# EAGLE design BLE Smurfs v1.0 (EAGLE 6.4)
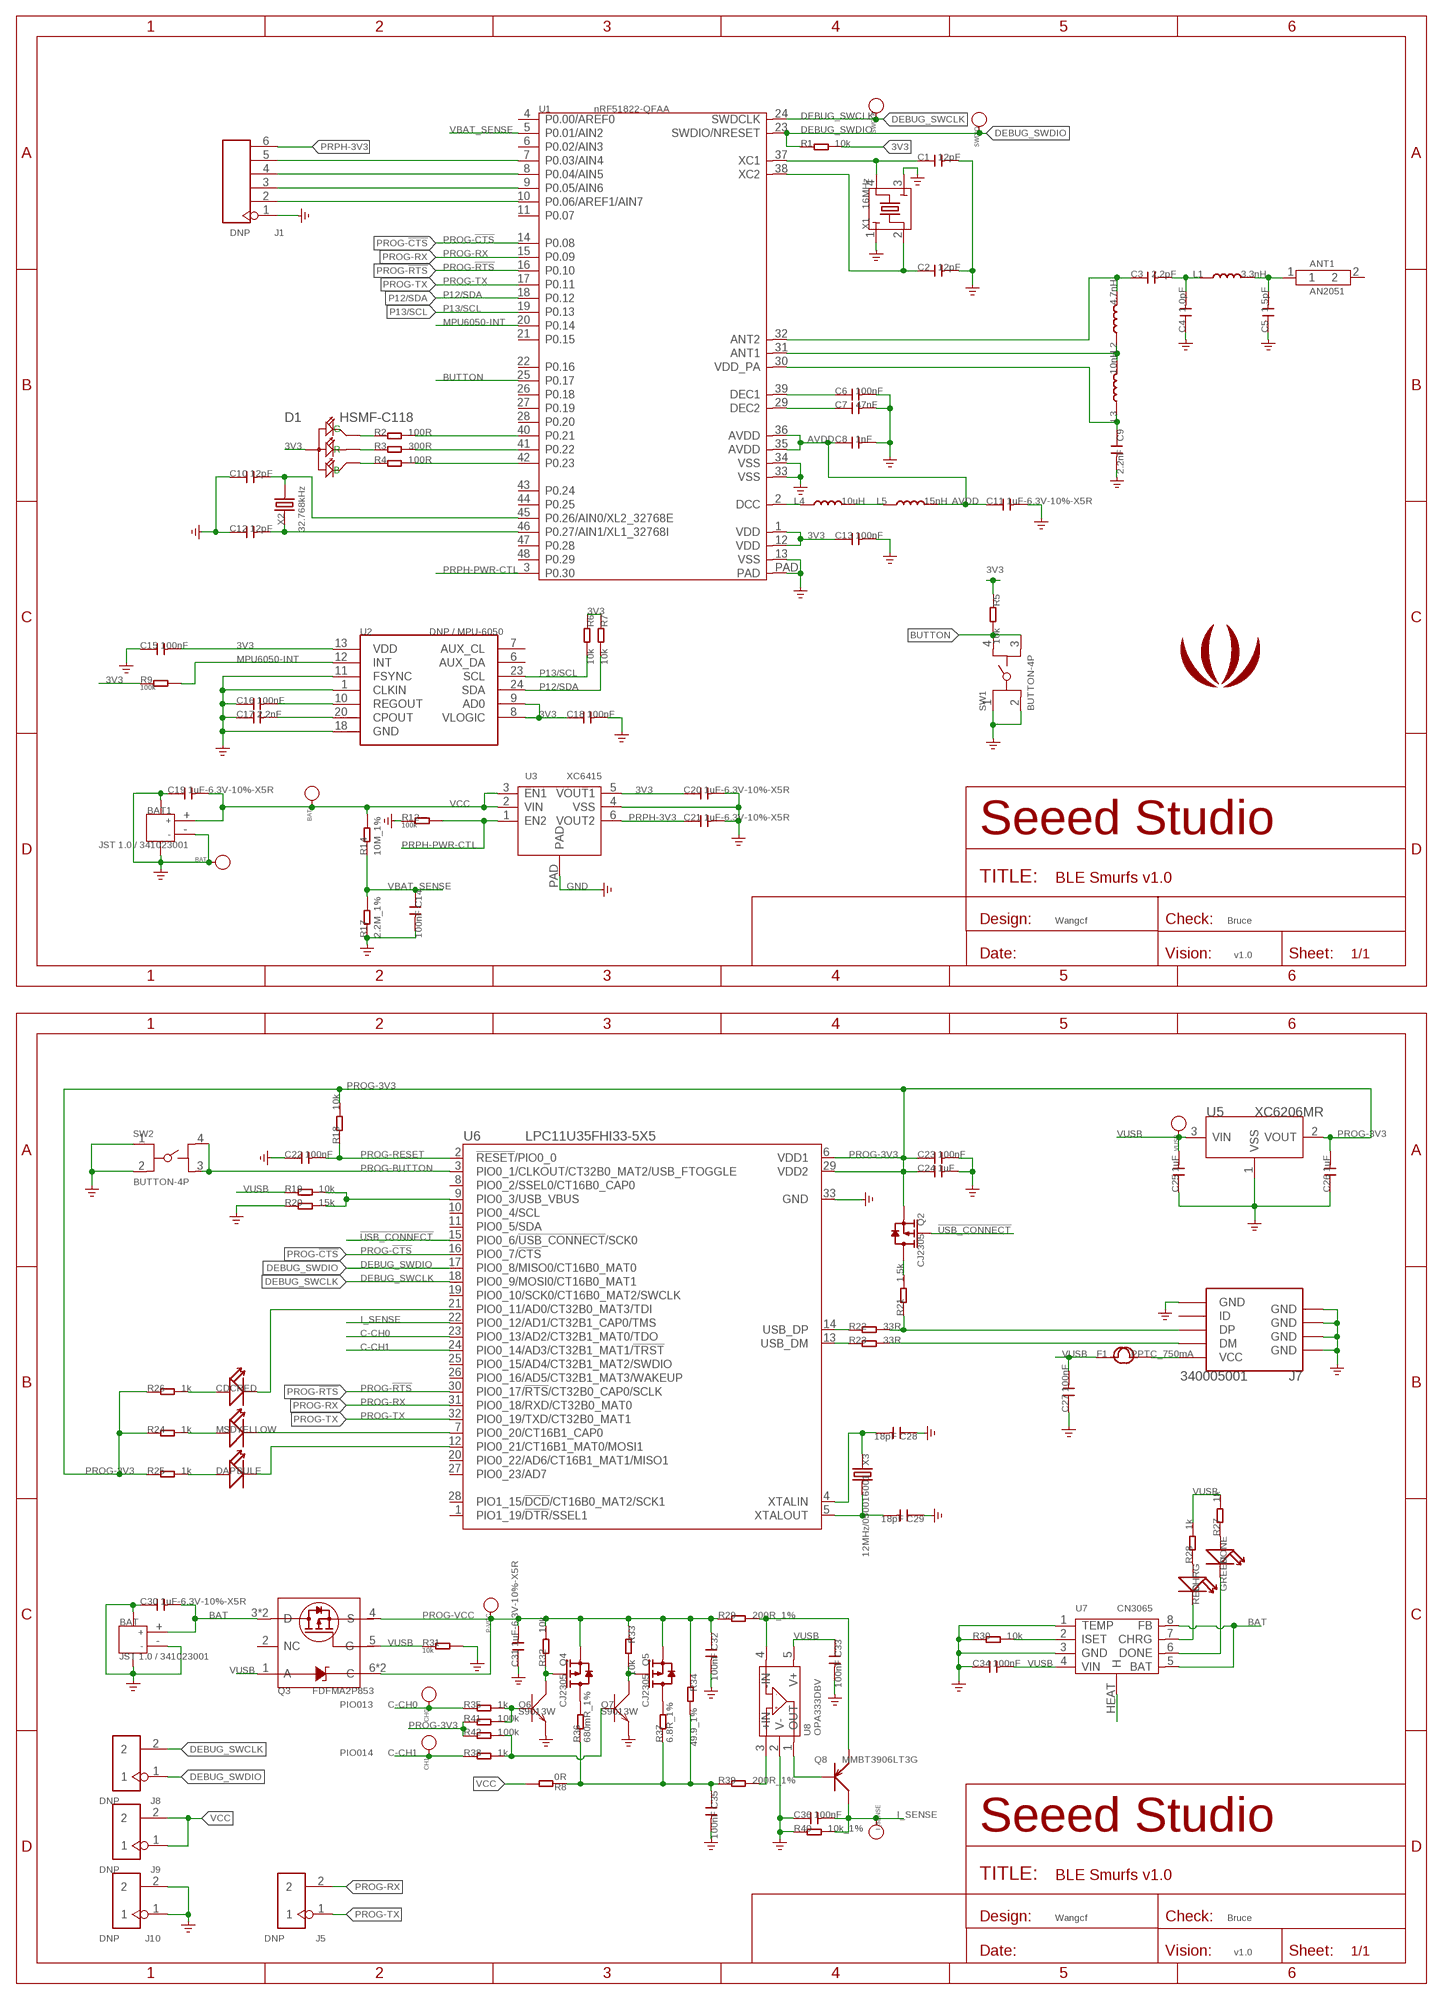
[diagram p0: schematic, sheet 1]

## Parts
ANT1  AN2051  ANTENNA-2.4GHZ-0.5DBI'AN2051'  [2P-SMD-L5.05*W.02*H1.07MM]
BAT  JST 1.0 / 341023001  JACK-JST-2P-SMD-PW'1.0'  [JST-SMD-2P-1.0-90D]
BAT1  JST 1.0 / 341023001  JACK-JST-2P-SMD-PW'1.0'  [JST-SMD-2P-1.0-90D]
BAT+  BAT+  PAD-TEST-POINT'4080'  [PAD_4080]
BAT-  BAT-  PAD-TEST-POINT'4080'  [PAD_4080]
C1  12pF  C-0402  [C0402]
C2  12pF  C-0402  [C0402]
C3  2.2pF  C-0402  [C0402]
C4  1.0pF  C-0402  [C0402]
C5  1.5pF  C-0402  [C0402]
C6  100nF  C-0402  [C0402]
C7  47nF  C-0402  [C0402]
C8  1nF  C-0402  [C0402]
C9  2.2nF  C-0402  [C0402]
C10  12pF  C-0402  [C0402]
C11  1uF-6.3V-10%-X5R  C-0402  [C0402]
C12  12pF  C-0402  [C0402]
C13  100nF  C-0402  [C0402]
C14  100nF  C-0402  [C0402]
C15  100nF  C-0402  [C0402]
C16  100nF  C-0402  [C0402]
C17  2.2nF  C-0402  [C0402]
C18  100nF  C-0402  [C0402]
C19  1uF-6.3V-10%-X5R  C-0402  [C0402]
C20  1uF-6.3V-10%-X5R  C-0402  [C0402]
C21  1uF-6.3V-10%-X5R  C-0402  [C0402]
C22  100nF  C-0402  [C0402]
C23  100nF  C-0402  [C0402]
C24  1uF  C-0402  [C0402]
C25  1uF  C-0402  [C0402]
C26  1uF  C-0402  [C0402]
C27  100nF  C-0402  [C0402]
C28  18pF  C-0402  [C0402]
C29  18pF  C-0402  [C0402]
C30  1uF-6.3V-10%-X5R  C-0402  [C0402]
C31  1uF-6.3V-10%-X5R  C-0402  [C0402]
C32  100nF  C-0402  [C0402]
C33  100nF  C-0402  [C0402]
C34  100nF  C-0402  [C0402]
C35  100nF  C-0402  [C0402]
C36  100nF  C-0402  [C0402]
CDC  RED  LED'0603'  [LED-0603]
CH0  CH0  PAD-TEST-POINT'4545'  [TP_4545]
CH1  CH1  PAD-TEST-POINT'4545'  [TP_4545]
CHRG  RED  LED'0603'  [LED-0603]
D1  HSMF-C118  LED-ARGB-4P-1210  [LED-4P-1210-3.0X2.54]
DAP  BULE  LED'0603'  [LED-0603]
DONE  GREEN  LED'0603'  [LED-0603]
F1  PPTC_750mA  FUSE'1206'  [F1206]
I_SENSE  I_SENSE  PAD-TEST-POINT'4545'  [TP_4545]
J1  DNP  HEADER-6P-60/35MIL  [6P-2.54-60/35MIL]
J5  DNP  HEADER-2P-65/35MIL  [2P-2.54-65/35MIL]
J7  340005001  USB-MINIUSB-5P-MICRO  [MICRO-USB]
J8  DNP  HEADER-2P-65/35MIL  [2P-2.54-65/35MIL]
J9  DNP  HEADER-2P-65/35MIL  [2P-2.54-65/35MIL]
J10  DNP  HEADER-2P-65/35MIL  [2P-2.54-65/35MIL]
L1  3.3nH  L'0402'  [L0402]
L2  4.7nH  L'0402'  [L0402]
L3  10nH  L'0402'  [L0402]
L4  10uH  L'0603'  [L0603]
L5  15nH  L'0402'  [L0402]
MSD  YELLOW  LED'0603'  [LED-0603]
P-VCC  P_VCC  PAD-TEST-POINT'4545'  [TP_4545]
Q2  CJ2305  MOSFET-P'SI2323CDS/SI2305DS<BR>'  [SOT23]
Q3  FDFMA2P853  [6P-SMD-W/-HEAT]
Q4  CJ2305  MOSFET-P'SI2323CDS/SI2305DS<BR>'  [SOT23]
Q5  CJ2305  MOSFET-P'SI2323CDS/SI2305DS<BR>'  [SOT23]
Q6  S9013W  TRANSISTOR-NPN-SOT323  [SOT323]
Q7  S9013W  TRANSISTOR-NPN-SOT323  [SOT323]
Q8  MMBT3906LT3G  TRANSISTOR-PNP-SOT23  [SOT23]
R1  10k  R-0402  [R0402]
R2  100R  R-0402  [R0402]
R3  300R  R-0402  [R0402]
R4  100R  R-0402  [R0402]
R5  10k  R-0402  [R0402]
R6  10k  R-0402  [R0402]
R7  10k  R-0402  [R0402]
R8  0R  R-0603  [R0603]
R9  100k  R-0402  [R0402]
R12  100k  R-0402  [R0402]
R14  10M_1%  R-0402  [R0402]
R17  2.2M_1%  R-0402  [R0402]
R18  10k  R-0402  [R0402]
R19  10k  R-0402  [R0402]
R20  15k  R-0402  [R0402]
R21  1.5k  R-0402  [R0402]
R22  33R  R-0402  [R0402]
R23  33R  R-0402  [R0402]
R24  1k  R-0402  [R0402]
R25  1k  R-0402  [R0402]
R26  1k  R-0402  [R0402]
R27  1k  R-0402  [R0402]
R28  1k  R-0402  [R0402]
R29  200R_1%  R-0402  [R0402]
R30  10k  R-0402  [R0402]
R31  10k  R-0402  [R0402]
R32  10k  R-0402  [R0402]
R33  10k  R-0402  [R0402]
R34  49.9_1%  R-0603  [R0603]
R35  1k  R-0402  [R0402]
R36  680mR_1%  R-0603  [R0603]
R37  6.8R_1%  R-0603  [R0603]
R38  1k  R-0402  [R0402]
R39  200R_1%  R-0402  [R0402]
R40  10k_1%  R-0402  [R0402]
R41  100k  R-0402  [R0402]
R42  100k  R-0402  [R0402]
SW1  BUTTON-4P  [4P-SMD-L4.45*W3.22*H2.5MM]
SW2  BUTTON-4P  [4P-SMD-L4.45*W3.22*H2.5MM]
SWCLK  SWDCLK  PAD-TEST-POINT'4080'  [PAD_4080]
SWDIO  SWDIO  PAD-TEST-POINT'4080'  [PAD_4080]
U1  nRF51822-QFAA  NRF51822  [QFN48-6X6MM]
U2  DNP / MPU-6050  MPU-6050‘’  [QFN24]
U3  XC6415  [USP-6C]
U5  XC6206MR  [SOT23]
U6  LPC11U35FHI33-5X5  [HVQFN33]
U7  CN3065  PMIC-CN3065-DFN8  [DFN-8]
U8  OPA333DBV  [SOT23-5]
U$59  LOGO-SEEEDSTUDIO-SMALL-SILK  [SMALL_SEEED_LOGO]
VUSB  VUSB  PAD-TEST-POINT'4545'  [TP_4545]
X1  16MHz  CRYSTAL'-2520'  [2520]
X2  32.768kHz  CRYSTAL-3215  [2P-SMD-3.2X1.5]
X3  12MHz/050016001  CRYSTAL'5032'  [2P-SMD-5X3.2]

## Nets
3V3: C13.1 C15.2 C18.1 C20.1 D1.1(+) R1.2 R5.1 R6.1 R7.1 R9.1 U1.1(VDD) U1.12(VDD) U2.8(VLOGIC) U2.9(AD0) U2.13(VDD) U3.5(VOUT1)
!USB_CONNECT: Q2.1(G) U6.15(PIO0_6/!USB_CONNECT!/SCK0)
AVDD: C8.1 C11.1 L5.2 U1.35(AVDD) U1.36(AVDD)
BAT: BAT.+ C30.2 Q3.3(D) Q3.P2(D) U7.5(BAT) U7.8(FB)
BUTTON: R5.2 SW1.3 SW1.4 U1.25(P0.17)
C-CH0: CH0.T R35.1 U6.23(PIO0_13/AD2/CT32B1_MAT0/TDO)
C-CH1: CH1.T R38.1 U6.24(PIO0_14/AD3/CT32B1_MAT1/!TRST!)
CHRG: CHRG.- U7.7(CHRG)
CHRG-DONE: DONE.- U7.6(DONE)
DCC: L4.1 U1.2(DCC)
DEBUG_SWCLK: J8.2 SWCLK.1(T) U1.24(SWDCLK) U6.18(PIO0_9/MOSI0/CT16B0_MAT1)
DEBUG_SWDIO: J8.1 R1.1 SWDIO.1(T) U1.23(SWDIO/NRESET) U6.17(PIO0_8/MISO0/CT16B0_MAT0)
GND: BAT1.3 BAT1.4 BAT1.- BAT-.1(T) BAT.3 BAT.4 BAT.- C1.2 C2.2 C4.1 C5.1 C6.2 C7.2 C8.2 C9.2 C10.1 C11.2 C12.1 C13.2 C14.2 C15.1 C16.1 C17.1 C18.2 C19.1 C20.2 C21.2 C22.1 C23.2 C24.2 C25.1 C26.1 C27.1 C28.1 C29.1 C30.1 C31.1 C32.2 C33.2 C34.1 C35.2 C36.1 J1.1 J7.5(GND) J7.S1(GND) J7.S2(GND) J7.S3(GND) J7.S4(GND) J7.S5(GND) J7.S6(GND) J10.1 J10.2 Q6.2(E) Q7.2(E) R12.1 R17.1 R20.1 R30.1 R31.2 R40.1 SW1.1 SW1.2 SW2.1 SW2.2 U1.13(VSS) U1.33(VSS) U1.34(VSS) U1.PAD U2.1(CLKIN) U2.11(FSYNC) U2.18(GND) U3.4(VSS) U3.PAD U5.1(VSS) U6.33(GND) U7.1(TEMP) U7.3(GND) U8.2(V-) X1.1 X1.3 ; supply symbol labelled GND_POWER
I_SENSE: C36.2 I_SENSE.T Q8.3(C) R40.2 U6.22(PIO0_12/AD1/CT32B1_CAP0/TMS)
ISET: R30.2 U7.2(ISET)
MPU6050-INT: R9.2 U1.20(P0.14) U2.12(INT)
N$1: Q8.2(E) R29.2 U8.4(-IN)
N$2: C29.2 U6.5(XTALOUT) X3.2
N$3: D1.3(G) R2.1
N$4: C28.2 U6.4(XTALIN) X3.1
N$5: D1.2(R) R3.1
N$6: R22.1 U6.14(USB_DP)
N$7: R23.1 U6.13(USB_DM)
N$8: J7.3(DP) R21.1 R22.2
N$9: Q4.1(G) Q6.3(C) R32.1
N$11: J7.2(DM) R23.2
N$12: C10.2 U1.45(P0.26/AIN0/XL2_32768E) X2.2
N$13: C12.2 U1.46(P0.27/AIN1/XL1_32768I) X2.1
N$14: C1.1 U1.37(XC1) X1.4
N$15: C2.1 U1.38(XC2) X1.2
N$16: CDC.- U6.21(PIO0_11/AD0/CT32B0_MAT3/TDI)
N$17: U7.HEAT(H)
N$19: C16.2 U2.10(REGOUT)
N$20: C6.1 U1.39(DEC1)
N$21: C17.2 U2.20(CPOUT)
N$25: C7.1 U1.29(DEC2)
N$26: C3.1 L2.2 U1.32(ANT2)
N$28: L2.1 L3.2 U1.31(ANT1)
N$29: C9.1 L3.1 U1.30(VDD_PA)
N$30: C3.2 C4.2 L1.1
N$31: ANT1.1 C5.2 L1.2
N$32: L4.2 L5.1
N$39: Q2.3(D) R21.2
N$40: F1.2 J7.1(VCC)
N$41: R19.2 R20.2 U6.9(PIO0_3/USB_VBUS)
N$42: CDC.+ R26.2
N$43: DAP.+ R25.2
N$44: MSD.+ R24.2
N$46: MSD.- U6.7(PIO0_20/CT16B1_CAP0)
N$47: DAP.- U6.12(PIO0_21/CT16B1_MAT0/MOSI1)
N$78: D1.4(B) R4.1
N$79: Q8.1(B) U8.1(OUT)
N$80: R39.2 U8.3(+IN)
N$81: Q5.3(D) R37.2
N$82: Q4.3(D) R36.2
N$83: Q6.1(B) R35.2 R41.2
N$84: Q5.1(G) Q7.3(C) R33.2
N$85: Q7.1(B) R38.2 R42.2
N$86: DONE.+ R27.1
N$87: CHRG.+ R28.1
N$88: R2.2 U1.40(P0.21)
N$89: R3.2 U1.41(P0.22)
N$90: R4.2 U1.42(P0.23)
N$93: J1.2 U1.10(P0.06/AREF1/AIN7)
N$94: J1.3 U1.9(P0.05/AIN6)
N$95: J1.4 U1.8(P0.04/AIN5)
N$96: J1.5 U1.7(P0.03/AIN4)
N$98: C35.1 R8.1 R34.2 R36.1 R37.1 R39.1
P12/SDA: R7.2 U1.18(P0.12) U2.24(SDA)
P13/SCL: R6.2 U1.19(P0.13) U2.23(SCL)
PROG-3V3: C23.1 C24.1 C26.2 Q2.2(S) R18.2 R24.1 R25.1 R26.1 R41.1 R42.1 U5.2(VOUT) U6.6(VDD1) U6.29(VDD2)
PROG-!CTS: U1.14(P0.08) U6.16(PIO0_7/!CTS!)
PROG-!RTS: U1.16(P0.10) U6.30(PIO0_17/!RTS!/CT32B0_CAP0/SCLK)
PROG-BUTTON: SW2.3 SW2.4 U6.3(PIO0_1/CLKOUT/CT32B0_MAT2/USB_FTOGGLE)
PROG-RESET: C22.2 R18.1 U6.2(!RESET!/PIO0_0)
PROG-RX: J5.2 U1.15(P0.09) U6.31(PIO0_18/RXD/CT32B0_MAT0)
PROG-TX: J5.1 U1.17(P0.11) U6.32(PIO0_19/TXD/CT32B0_MAT1)
PROG-VCC: C31.2 C32.1 P-VCC.T Q3.4(S) Q3.6(C) Q3.P1(C) Q4.2(S) Q5.2(S) R29.1 R32.2 R33.1 R34.1
PRPH-3V3: C21.1 J1.6 U3.6(VOUT2)
PRPH-PWR-CTL: R12.2 U1.3(P0.30) U3.1(EN2)
VBAT_SENSE: C14.1 R14.1 R17.2 U1.5(P0.01/AIN2)
VCC: BAT1.+ BAT+.1(T) C19.2 J9.1 J9.2 R8.2 R14.2 U3.2(VIN) U3.3(EN1)
VUSB: C25.2 C27.2 C33.1 C34.2 F1.1 Q3.1(A) Q3.5(G) R19.1 R27.2 R28.2 R31.1 U5.3(VIN) U7.4(VIN) U8.5(V+) VUSB.T
Unconnected: ANT1.2 J7.4(ID) Q3.2(NC) U1.4(P0.00/AREF0) U1.6(P0.02/AIN3) U1.11(P0.07) U1.21(P0.15) U1.22(P0.16) U1.26(P0.18) U1.27(P0.19) U1.28(P0.20) U1.43(P0.24) U1.44(P0.25) U1.47(P0.28) U1.48(P0.29) U2.6(AUX_DA) U2.7(AUX_CL) U6.1(PIO1_19/!DTR!/SSEL1) U6.8(PIO0_2/SSEL0/CT16B0_CAP0) U6.10(PIO0_4/SCL) U6.11(PIO0_5/SDA) U6.19(PIO0_10/SCK0/CT16B0_MAT2/SWCLK) U6.20(PIO0_22/AD6/CT16B1_MAT1/MISO1) U6.25(PIO0_15/AD4/CT32B1_MAT2/SWDIO) U6.26(PIO0_16/AD5/CT32B1_MAT3/WAKEUP) U6.27(PIO0_23/AD7) U6.28(PIO1_15/!DCD!/CT16B0_MAT2/SCK1)

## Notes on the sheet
- Wangcf | Bruce
- v1.0
- PIO013
- PIO014
- Wangcf | Bruce
- v1.0

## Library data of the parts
ANT1 = Connector:ANTENNA-2.4GHZ-0.5DBI: AN2051
BAT BAT1 = Connector :JACK-JST-2P-SMD-PW
BAT+ BAT- SWCLK SWDIO = Discrete:PAD-TEST-POINT
C1-C36 = Discrete:C*: Ceramic Capacitors
CDC CHRG DAP DONE MSD = Discrete:LED*
CH0 CH1 I_SENSE P-VCC VUSB = Discrete:PAD-TEST-POINT; PARTNO: DNP
D1 = Discrete:LED-ARGB*-4P
F1 = Discrete:FUSE
J1 = Connector:HEADER-6P
J5 J8-J10 = Connector:HEADER-2P
J7 = Connector :USB-MINIUSB-5P
L1-L5 = Discrete:L*
Q2 Q4 Q5 = Discrete:MOSFET-P
Q3 = template:FDFMA2P853: Integrated P-Channel Power Trench MOSFET and Schottky Diode
Q6 Q7 = Discrete:TRANSISTOR-NPN*: NPN audion
Q8 = Discrete:TRANSISTOR-PNP*: PNP audion
R1-R9 R12 R14 R17-R42 = Discrete:R*
SW1 SW2 = template:BUTTON-4P
U1 = AMLib:NRF51822: Multi-protocol Blutooth 4.0 low energy /2. GHz RF SoC
U2 = template:MPU-6050
U3 = template :XC6415: Dual LDO Regulator with ON/OFF Switch
U5 = IC:XC6206: LOW ESR Cap.Compatible Positive Voltage Regulators
U6 = AMLib:LPC11U35FHI33
U7 = IC-new:PMIC-CN3065: 310030101
U8 = IC:OPA333: 1.8V,Micro power CMOS oprational amplifiers Zero-Drift Series http://www.ti.com.cn/cn/lit/ds/symlink/opa333.pdf
U$59 = Logo:LOGO-SEEEDSTUDIO; PARTNO: DNP
X1 = AMLib:CRYSTAL
X2 X3 = Discrete:CRYSTAL*: CRYSTAL

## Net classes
0 default: width 0.102 mm, drill 0.203 mm, clearance 0.102 mm

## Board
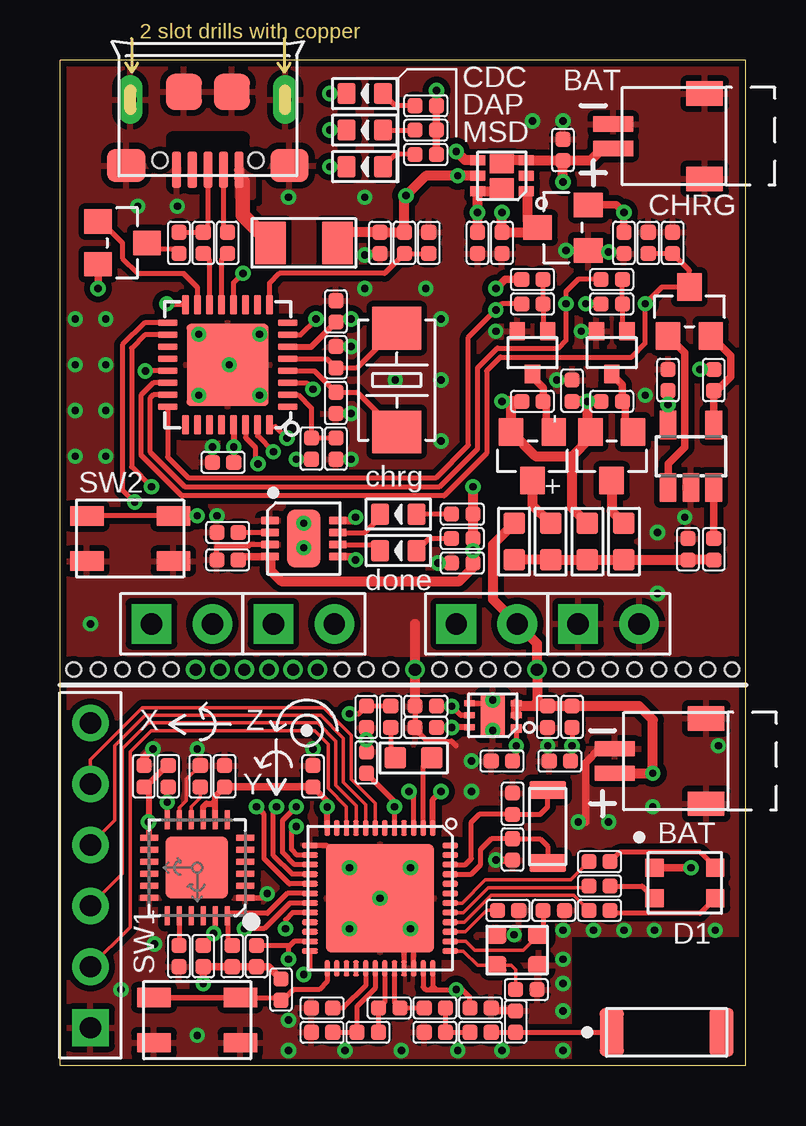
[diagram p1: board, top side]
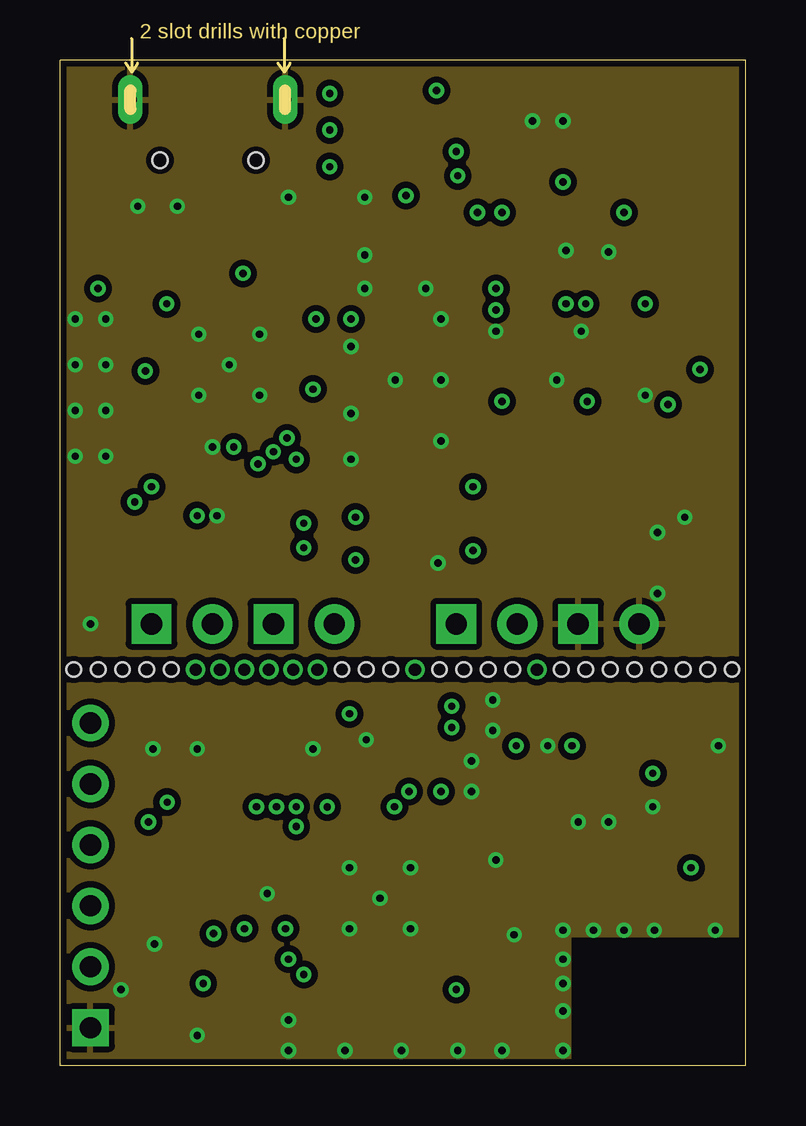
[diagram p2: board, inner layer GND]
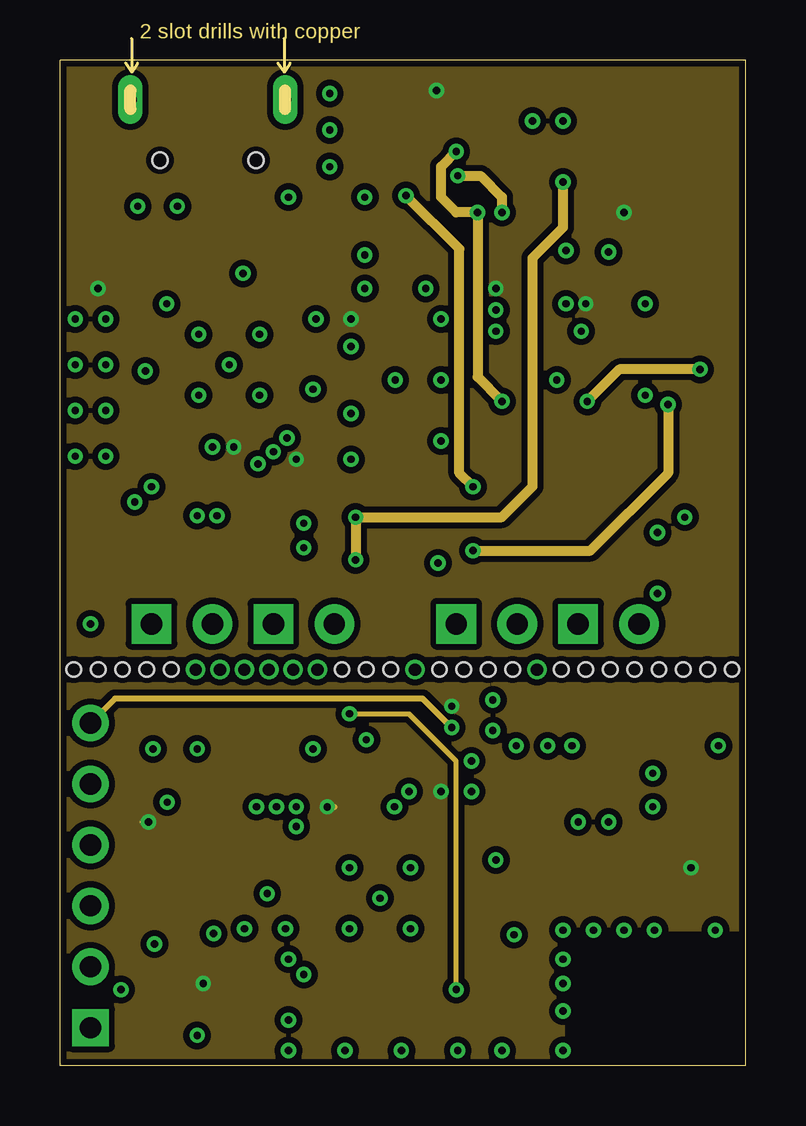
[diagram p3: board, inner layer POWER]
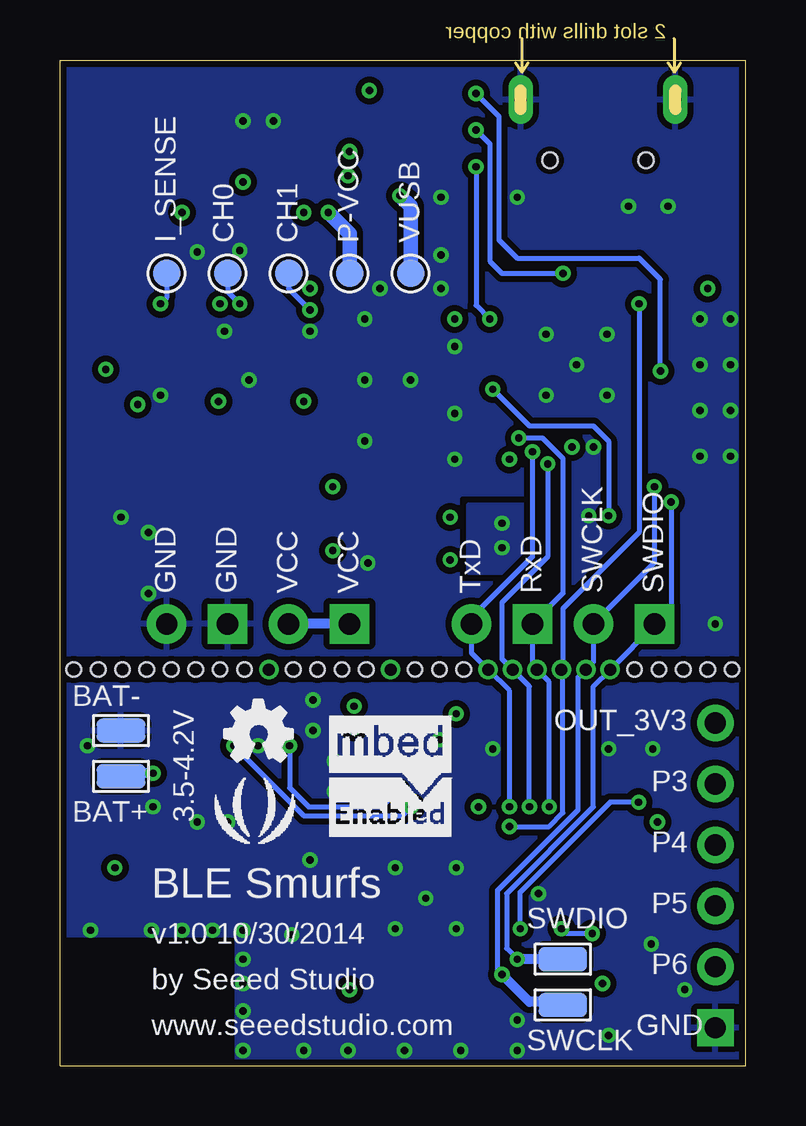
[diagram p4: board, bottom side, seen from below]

Size 28.57 x 41.91 mm. Coordinates in mm from the lower left corner, seen from the top.
Outline: 0,0 0,41.91 28.57,41.91 28.57,0 0,0
Copper layers (1*2*15*16): Top 0.035mm / dielectric 0.2mm / GND 0.0175mm / dielectric 0.3mm / POWER 0.0175mm / dielectric 0.2mm / Bottom 0.035mm
Design rules "default": minimum track width 6mil, minimum drill 12mil, track to track 6mil, track to pad 6mil, pad to pad 6mil, via to via 6mil, smd to smd 0mil, copper to edge 6mil, drill to drill 10mil, minimum pad ring 6mil, minimum via ring 6mil, stop-mask expansion 2mil, vias tented up to drill 25mil, thermal gap 10mil
Holes 0.6 mm at 28,16.51 26.99,16.51 25.97,16.51 24.96,16.51 23.94,16.51 22.92,16.51 21.91,16.51 20.89,16.51 18.86,16.51 17.84,16.51 16.83,16.51 15.81,16.51 13.78,16.51 12.76,16.51 11.75,16.51 4.64,16.51 3.62,16.51 2.6,16.51 1.59,16.51 0.57,16.51

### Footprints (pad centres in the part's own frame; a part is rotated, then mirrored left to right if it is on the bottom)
2P-SMD-L5.05*W.02*H1.07MM = smd 1.016 x 2.032: 1 -2.286,0; 2 2.286,0
JST-SMD-2P-1.0-90D = smd 1.524 x 1.016: 3 -3.429,1.778; 4 -3.429,-1.778 | smd 1.651 x 0.635: + 0.381,0.508; - 0.381,-0.508
PAD_4080 = smd 2.032 x 1.016: 1 0,0
C0402 = smd 0.635 x 0.635: 1 -0.445,0; 2 0.445,0
LED-0603 = smd 0.762 x 0.889: + -0.762,0; - 0.762,0
TP_4545 = smd 1.143 x 1.143: T 0,0
LED-4P-1210-3.0X2.54 = smd 0.762 x 0.762: 1 -0.635,-1.27; 2 0.635,-1.27; 3 0.635,1.27; 4 -0.635,1.27
F1206 = smd 1.27 x 1.778: 1 -1.397,0; 2 1.397,0
6P-2.54-60/35MIL = drill 0.889 pad 1.524 square: 1 0,6.35 | drill 0.889 pad 1.524: 2 0,3.81; 3 0,1.27; 4 0,-1.27; 5 0,-3.81; 6 0,-6.35
2P-2.54-65/35MIL = drill 0.889 pad 1.651 square: 1 0,1.27 | drill 0.889 pad 1.651: 2 0,-1.27
MICRO-USB = smd 0.381 x 1.524: 1 -1.3,-0.25; 2 -0.65,-0.25; 3 0,-0.25; 4 0.65,-0.25; 5 1.3,-0.25 | smd 1.6 x 1.397: S1 -3.4,-0.427; S6 3.4,-0.427 | drill 0.508 pad 1.016 long: S2 -3.226,-3.175; S5 3.226,-3.175 | smd 1.5 x 1.5: S3 -1,-3.5; S4 1,-3.5 | hole 0.635: -2,-0.65; 2,-0.65
L0402 = smd 0.635 x 0.635: 1 -0.445,0; 2 0.445,0
L0603 = smd 0.889 x 0.889: 1 -0.762,0; 2 0.762,0
SOT23 = smd 1.016 x 1.143: 1 -0.889,-1.016; 2 0.889,-1.016; 3 0,1.016
6P-SMD-W/-HEAT = smd 0.42 x 0.62: 1 -0.65,-1.015; 2 0,-1.015; 3 0.65,-1.015; 4 0.65,1.015; 5 0,1.015; 6 -0.65,1.015 | smd 0.8 x 1: P1 -0.508,0; P2 0.5,0
SOT323 = smd 0.635 x 0.762: 1 -0.635,-0.889; 2 0.635,-0.889; 3 0,0.889
R0402 = smd 0.635 x 0.635: 1 -0.445,0; 2 0.445,0
R0603 = smd 0.889 x 0.889: 1 -0.762,0; 2 0.762,0
4P-SMD-L4.45*W3.22*H2.5MM = smd 1.4 x 0.8: 1 -1.8,-0.94; 2 1.8,-0.94; 3 1.8,0.94; 4 -1.8,0.94
QFN48-6X6MM = smd 0.23 x 0.65: 1 -2.2,-2.925; 2 -1.8,-2.925; 3 -1.4,-2.925; 4 -1,-2.925; 5 -0.6,-2.925; 6 -0.2,-2.925; 7 0.2,-2.925; 8 0.6,-2.925; 9 1,-2.925; 10 1.4,-2.925; 11 1.8,-2.925; 12 2.2,-2.925; 25 2.2,2.925; 26 1.8,2.925; 27 1.4,2.925; 28 1,2.925; 29 0.6,2.925; 30 0.2,2.925; 31 -0.2,2.925; 32 -0.6,2.925; 33 -1,2.925; 34 -1.4,2.925; 35 -1.8,2.925; 36 -2.2,2.925 | smd 0.65 x 0.23: 13 2.925,-2.2; 14 2.925,-1.8; 15 2.925,-1.4; 16 2.925,-1; 17 2.925,-0.6; 18 2.925,-0.2; 19 2.925,0.2; 20 2.925,0.6; 21 2.925,1; 22 2.925,1.4; 23 2.925,1.8; 24 2.925,2.2; 37 -2.925,2.2; 38 -2.925,1.8; 39 -2.925,1.4; 40 -2.925,1; 41 -2.925,0.6; 42 -2.925,0.2; 43 -2.925,-0.2; 44 -2.925,-0.6; 45 -2.925,-1; 46 -2.925,-1.4; 47 -2.925,-1.8; 48 -2.925,-2.2 | smd 4.5 x 4.5: PAD 0,0
QFN24 = smd 0.8 x 0.26: 1 -2,1.25; 2 -2,0.75; 3 -2,0.25; 4 -2,-0.25; 5 -2,-0.75; 6 -2,-1.25; 13 2,-1.25; 14 2,-0.75; 15 2,-0.25; 16 2,0.25; 17 2,0.75; 18 2,1.25 | smd 0.26 x 0.8: 7 -1.25,-2; 8 -0.75,-2; 9 -0.25,-2; 10 0.25,-2; 11 0.75,-2; 12 1.25,-2; 19 1.25,2; 20 0.75,2; 21 0.25,2; 22 -0.25,2; 23 -0.75,2; 24 -1.25,2 | smd 2.6 x 2.6: E 0.02,-0.01
USP-6C = smd 0.45 x 0.35: 1 -0.975,0.55 | smd 0.45 x 0.25: 2 -0.975,0; 3 -0.975,-0.5; 4 0.975,-0.5; 5 0.975,0; 6 0.975,0.5 | smd 1 x 1.8: PAD 0,0
SOT23' = smd 1.016 x 1.2: 1 -0.95,-1.06; 2 0.95,-1.06; 3 0,1.06
HVQFN33 = smd 0.813 x 0.279: 1 -2.5,1.75; 2 -2.5,1.25; 3 -2.5,0.75; 4 -2.5,0.25; 5 -2.5,-0.25; 6 -2.5,-0.75; 7 -2.5,-1.25; 8 -2.5,-1.75; 17 2.5,-1.75; 18 2.5,-1.25; 19 2.5,-0.75; 20 2.5,-0.25; 21 2.5,0.25; 22 2.5,0.75; 23 2.5,1.25; 24 2.5,1.75 | smd 0.279 x 0.813: 9 -1.75,-2.5; 10 -1.25,-2.5; 11 -0.75,-2.5; 12 -0.25,-2.5; 13 0.25,-2.5; 14 0.75,-2.5; 15 1.25,-2.5; 16 1.75,-2.5; 25 1.75,2.5; 26 1.25,2.5; 27 0.75,2.5; 28 0.25,2.5; 29 -0.25,2.5; 30 -0.75,2.5; 31 -1.25,2.5; 32 -1.75,2.5 | smd 3.429 x 3.429: 33 0,0
DFN-8 = smd 0.3 x 0.727: 1 -0.75,-1.413; 2 -0.25,-1.413; 3 0.25,-1.413; 4 0.75,-1.413; 5 0.75,1.413; 6 0.25,1.413; 7 -0.25,1.413; 8 -0.75,1.413 | smd 2.413 x 1.397: HEAT 0,0
SOT23-5 = smd 0.69 x 1.2: 1 -0.95,-1.3; 2 0,-1.3; 3 0.95,-1.3; 4 0.95,1.3; 5 -0.95,1.3
2520 = smd 0.889 x 0.762: 1 -0.889,0.635; 2 -0.889,-0.635; 3 0.889,-0.635; 4 0.889,0.635
2P-SMD-3.2X1.5 = smd 0.762 x 1.524: 1 -1.524,0; 2 1.524,0
2P-SMD-5X3.2 = smd 1.778 x 2.032: 1 -2.159,0; 2 2.159,0

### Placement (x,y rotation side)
ANT1  25.27,1.4 0 top
BAT  23.43,38.73 180 top
BAT1  23.5,12.7 180 top
BAT+  26.03,12.06 0 bottom
BAT-  26.03,13.97 0 bottom
C1  19.43,3.17 0 top
C2  20.57,6.48 0 top
C3  15.62,2.41 0 top
C4  15.62,1.4 0 top
C5  18.99,1.84 270 top
C6  18.67,6.48 0 top
C7  10.92,2.41 180 top
C8  17.53,2.41 0 top
C9  10.92,1.4 180 top
C10  18.86,9.02 90 top
C11  12.76,14.54 270 top
C12  18.86,10.92 270 top
C13  10.54,12.06 90 top
C14  12.76,12.64 90 top
C15  3.49,12.06 270 top
C16  5.84,12.06 270 top
C17  4.95,4.57 90 top
C18  6.86,12.06 90 top
C19  20.32,14.54 90 top
C20  15.24,14.99 180 top
C21  15.24,14.1 180 top
C22  11.49,25.72 90 top
C23  11.49,31.43 90 top
C24  6.79,25.15 180 top
C25  18.41,34.29 90 top
C26  23.5,34.29 90 top
C27  13.33,34.29 90 top
C28  11.49,27.62 90 top
C29  11.49,29.53 270 top
C30  20.95,38.16 270 top
C31  17.4,34.29 90 top
C32  21.34,28.13 90 top
C33  25.34,28.57 90 top
C34  6.98,21.08 0 top
C35  26.16,21.53 90 top
C36  25.53,34.29 270 top
CDC  12.7,40.51 180 top
CH0  21.59,33.02 0 bottom
CH1  19.05,33.02 0 bottom
CHRG  14.1,22.99 180 top
D1  26.03,7.62 270 top
DAP  12.7,38.99 180 top
DONE  14.1,21.46 180 top
F1  10.16,34.29 180 top
I_SENSE  24.13,33.02 0 bottom
J1  1.27,7.94 180 top
J5  10.16,18.41 90 top
J7  6.16,37.08 180 top
J8  5.08,18.41 90 top
J9  17.78,18.41 90 top
J10  22.86,18.41 90 top
L1  17.53,1.4 0 top
L2  13.72,2.41 0 top
L3  12.83,1.4 0 top
L4  14.73,12.83 180 top
L5  13.78,14.54 90 top
MSD  12.7,37.46 180 top
P-VCC  16.51,33.02 0 bottom
Q2  2.6,34.29 270 top
Q3  18.41,37.08 90 top
Q4  22.99,25.4 180 top
Q5  19.69,25.4 180 top
Q6  22.99,29.72 180 top
Q7  19.69,29.72 180 top
Q8  26.23,31.43 0 top
R1  8.19,4.57 270 top
R2  22.48,6.48 180 top
R3  22.48,7.49 180 top
R4  22.48,8.51 180 top
R5  9.21,3.17 270 top
R6  5.97,4.57 90 top
R7  7.18,4.57 90 top
R8  18.92,21.84 90 top
R9  4.51,12.06 270 top
R12  18.41,12.7 0 top
R14  21.34,14.54 90 top
R17  20.83,12.7 0 top
R18  10.48,25.72 270 top
R19  14.35,34.29 270 top
R20  15.37,34.29 270 top
R21  4.95,34.29 270 top
R22  5.97,34.29 90 top
R23  6.98,34.29 90 top
R24  15.24,37.97 180 top
R25  15.24,38.99 180 top
R26  15.24,40 180 top
R27  16.76,21.97 0 top
R28  16.76,22.99 0 top
R29  27.24,28.57 270 top
R30  6.98,22.22 0 top
R31  16.76,20.95 180 top
R32  22.99,27.69 180 top
R33  19.69,27.69 0 top
R34  21.97,21.84 270 top
R35  22.99,32.77 0 top
R36  23.5,21.84 90 top
R37  20.45,21.84 90 top
R38  19.69,31.75 0 top
R39  27.24,21.53 90 top
R40  24.51,34.29 270 top
R41  22.99,31.75 0 top
R42  19.69,32.77 0 top
SW1  5.72,1.9 0 top
SW2  2.92,21.97 0 top
SWCLK  7.62,2.54 180 bottom
SWDIO  7.62,4.45 180 bottom
U1  13.33,6.98 180 top
U2  5.72,8.25 180 top
U3  18.03,14.6 180 top
U5  XC6206MR  [SOT23']  20.95,34.92 90 top
U6  6.98,29.21 180 top
U7  10.16,21.97 270 top
U8  26.29,25.4 0 top
U$30  [OSHW_FILLX100_NOTEXT]  21.72,12.7 0 bottom
U$59  20.45,10.79 0 bottom
VUSB  13.97,33.02 0 bottom
X1  19.05,4.83 180 top
X2  20.32,9.97 270 top
X3  14.03,28.57 90 top

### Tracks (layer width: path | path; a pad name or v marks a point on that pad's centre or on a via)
3V3  (via drill 0.3 pad 0.64)
  Top 0.203: 3.72,11.72 3.65,11.72 | 4.38,12.32 4.38,12.38 R9.1 | 16.83,14.6 U3.5 16.7,14.6 v16.32,14.99 C20.1
  Top 0.254: U1.12 v11.13,10.79 11.13,11.03 C13.1 | U2.8 6.47,10.81 | 6.47,10.81 6.47,10.92 | 6.47,10.92 6.47,11.23 C18.1 | U2.9 5.97,10.79 6.1,10.92 6.35,10.92 | 6.35,10.92 6.47,10.92 | 6.35,10.92 6.41,10.99 | 6.47,10.81 6.35,10.92 | U2.13 3.72,10.19 | 3.72,10.19 3.72,11.72 3.72,11.78 4.25,12.32 4.38,12.32 | 3.72,10.19 v3.68,10.16 | U1.1 15.53,11.09 v15.88,11.43
  Top 0.305: C13.1 C18.1 | R1.2 R7.1 R6.1 v5.97,3.43 | R1.2 8.25,4.13 | D1.1 v26.29,8.25 | 3.65,11.72 3.59,11.72 C15.2 | R1.2 8.7,4.13 R5.1
  POWER 0.254: 11.43,10.79 | v3.68,10.16 3.43,10.16
  pour POWER (isolate 0.254): 0,0 20.95,0 20.95,5.71 29.84,5.71 29.84,15.87 0,15.87
!USB_CONNECT
  Top 0.203: Q2.1 1.71,35.18 2.6,34.29 2.6,33.66 3.24,33.02 5.14,33.02 5.73,32.43 U6.15
AVDD  (via drill 0.3 pad 0.64)
  Top 0.203: U1.35 15.13,3.28 15.24,3.17 15.43,3.17 | 15.43,3.17 15.49,3.17 | 15.49,3.17 15.68,3.17 | 15.68,3.17 v16.51,3.17 16.76,3.17 17.08,2.86 C8.1 | U1.36 15.53,3.32 | 15.53,3.28 15.53,3.22 15.49,3.17 | 15.53,3.32 15.53,3.28 | 15.53,3.28 15.43,3.17 | 15.53,3.32 15.68,3.17 | L5.2 C11.1 12.45,14.67 v12.06,14.67
  POWER 0.203: v16.51,3.17 16.51,12.7 14.54,14.67 v12.06,14.67
BAT  (via drill 0.3 pad 0.64)
  Top 0.254: C30.2 20.94,37.73
  Top 0.305: U7.8 12.18,22.72 v12.32,22.86 | U7.5 12.18,21.22 v12.32,21.08
  Top 0.406: Q3.P2 18.56,37.73 Q3.3 20.94,37.73 22.11,37.73 22.61,38.23 BAT.+ | v20.95,36.83 C30.2
  POWER 0.406: v20.95,36.83 20.95,34.92 19.69,33.66 19.69,24.13 18.41,22.86 v12.32,22.86 v12.32,21.08
BUTTON
  Top 0.203: SW1.3 SW1.4 9.09,2.84 R5.2 9.27,2.79 9.33,2.79 9.72,3.17 10.79,3.17 11.13,3.52 U1.25
C-CH0  (via drill 0.3 pad 0.64)
  Top 0.203: U6.23 3.89,27.96 3.75,27.81 3.75,25.59 5.21,24.13 15.82,24.13 17.4,25.71 17.4,29.08 18.22,29.91 20.76,29.91 21.08,30.23 v21.08,31.75 21.08,32.26 21.59,32.77 R35.1
  Bottom 0.203: 21.34,33.02 CH0.T 21.59,32.26 v21.08,31.75
C-CH1  (via drill 0.3 pad 0.64)
  Top 0.203: U6.24 4.48,25.36 5.33,24.51 15.67,24.51 17.02,25.86 17.02,30.35 v18.16,31.5 18.41,31.75 R38.1
  Bottom 0.203: CH1.T 19.05,32.38 v18.16,31.5
CHRG
  Top 0.203: U7.7 12.7,22.22 13.33,22.86 CHRG.-
CHRG-DONE
  Top 0.203: U7.6 13.08,21.72 DONE.-
DCC
  Top 0.203: U1.2 15.13,12.47 L4.1
DEBUG_SWCLK  (via drill 0.3 pad 0.64, 0.51 pad 0.76)
  Top 0.203: U1.24 10.41,4.06 v10.16,3.81 | U6.18 3.54,30.46 2.98,29.91 2.98,24.95 v3.81,24.13
  Bottom 0.203: v10.16,3.81 10.35,4 10.35,7.3 6.98,10.67 6.98,16.19 v6.67,16.51 6.35,16.83 J8.2 3.81,20.95 v3.81,24.13
  Bottom 0.406: SWCLK.1 8.25,2.54 8.25,2.67 9.02,2.67 v10.16,3.81
DEBUG_SWDIO  (via drill 0.3 pad 0.64, 0.51 pad 0.76)
  Top 0.203: U1.23 9.76,5.18 9.59,5.02 | 9.59,5.02 9.53,4.95 v9.53,4.45 | R1.1 9.59,5.02 | U6.17 3.53,30.96 2.6,30.03 2.6,24 v3.11,23.49
  Bottom 0.203: v9.53,4.45 9.97,4.89 9.97,7.18 6.35,10.79 6.35,15.81 v5.65,16.51 3.81,18.35 J8.1 3.11,19.11 v3.11,23.49
  Bottom 0.406: SWDIO.1 v9.53,4.45
GND  (via drill 0.3 pad 0.64, 0.51 pad 0.76)
  Top 0.152: U2.11 4.97,10.74 5.27,11.05 5.27,11.94 C16.1
  Top 0.203: U1.13 11.13,9.18 11.43,8.89 11.56,8.89 12.19,8.25 v12.06,8.25 | U1.33 14.33,5.35 | 14.33,5.35 13.97,5.71 | 14.73,5.08 U1.34 14.73,5.59 v14.6,5.71 14.33,5.45 14.33,5.35 | C16.1 5.78,12.51 | U2.1 8.47,7 v8.64,7.18 | U3.4 18.03,15.1 v18.03,15.24 | C20.2 14.8,14.16 | 14.8,14.16 14.86,14.1 | 14.8,14.16 14.8,14.03 15.3,13.52 16.32,13.52 16.51,13.33 | 6.6,21.72 | C34.1 6.54,21.66 6.6,21.72 | U7.3 7.94,21.72 7.87,21.65 6.67,21.65 6.6,21.72
  Top 0.305: C5.1 18.1,2.29 C8.2 | C10.1 v18.16,8.57 | C11.2 12.64,14.1 | 20.45,13.97 C19.1 | C15.1 3.49,12.83 v3.87,13.21 | C27.1 12.76,33.85 v12.7,33.78 | BAT1.- 22.48,13.21 21.91,12.64 21.91,10.16
  Top 0.406: C20.2 v14.8,16.51 14.8,18.41
  other vias: 17.14,11.43 18.16,30.61 20.95,2.29 20.95,3.43 20.95,4.45 20.95,5.65 22.22,5.65 23.5,5.65 24.76,5.65 27.31,5.65 20.32,13.33 18.03,13.97 21.59,10.16 22.86,10.16 24.7,10.79 18.92,5.46 13.33,6.98 14.6,8.25 12.06,5.71 5.72,1.27 2.54,3.17 7.05,29.21 5.78,27.94 8.32,27.94 8.32,30.48 5.78,30.48 6.35,25.78 21.72,30.61 26.03,22.86 13.97,28.57 15.88,28.57 15.88,31.11 12.13,29.97 6.54,22.92 20.7,28.57 15.88,26.03 5.72,13.21 4.89,35.81 3.24,35.81 24.89,22.22 24.89,19.68 9.53,1.9 12.13,27.18 12.13,25.27 12.76,13.59 17.14,12.7 10.54,13.21 9.53,0.63 11.87,0.63 14.22,0.63 16.57,0.63 18.41,0.63 20.95,0.63 15.75,20.95 21.08,33.97 22.86,33.91 12.7,32.38 9.53,36.2 12.7,36.2 20.95,39.37 19.69,39.37 15.24,32.38 24.38,27.94 3.94,5.08 27.43,13.33 0.63,31.11 1.91,31.11 0.63,29.21 1.91,29.21 0.63,27.3 1.91,27.3 0.63,25.4 1.91,25.4 1.27,18.41
  pour GND (isolate 0.254): 0,0 21.21,0 21.21,5.46 29.21,5.46 29.21,15.87 0,15.87
  pour GND (isolate 0.254): 0,17.14 29.21,17.14 29.21,41.91 0,41.91
  pour Top (isolate 0.254, rank 2): 0,17.14 28.57,17.14 28.57,41.91 0,41.91
  pour Bottom (isolate 0.254, rank 2): 0,17.14 28.57,17.14 28.57,41.91 0,41.91
  pour Top (isolate 0.254): 0,15.87 28.57,15.87 28.57,5.46 21.21,5.46 21.21,0 0,0
  pour Bottom (isolate 0.254): 0,15.87 28.57,15.87 28.57,5.46 21.21,5.46 21.21,0 0,0
I_SENSE  (via drill 0.3 pad 0.64)
  Top 0.203: U6.22 3.88,28.46 3.37,27.94 3.37,25.46 5.08,23.75 16,23.75 17.78,25.53 17.78,28.96 18.35,29.53 23.81,29.53 24.38,30.1 v24.38,31.75 25.08,32.45 Q8.3 26.22,33.15 C36.2 R40.2
  Bottom 0.203: I_SENSE.T 24.13,32 v24.38,31.75
ISET
  Top 0.203: U7.2 R30.2
MPU6050-INT  (via drill 0.3 pad 0.64)
  Top 0.203: U1.20 9.69,6.38 9.4,6.1 v9.4,5.71 | U2.12 v4.47,10.99 4.47,11.51
  Top 0.254: 4.47,11.51 4.47,11.58 R9.2
  Bottom 0.203: v4.47,10.99 5.65,10.99 9.4,7.24 v9.4,5.71
N$1
  Top 0.305: U8.4 R29.2 27.37,28.13 27.94,28.7 27.94,29.59 Q8.2
N$2
  Top 0.203: U6.5 11.12,29.46 C29.2 12.38,29.08 X3.2
N$3
  Top 0.203: D1.3 26.67,6.35 23.05,6.35 R2.1
N$4
  Top 0.203: U6.4 10.6,28.96 C28.2 12.38,28.07 X3.1
N$5
  Top 0.203: R3.1 24.26,7.49 D1.2
N$6
  Top 0.203: U6.14 6.23,33.58 R22.1
N$7
  Top 0.203: U6.13 6.73,33.6 R23.1
N$8
  Top 0.203: R21.1 R22.2 6.16,34.92 J7.3
N$9
  Top 0.305: Q6.3 23.43,28.38 R32.1 23.56,27.69 23.56,26.73 Q4.1
N$11
  Top 0.203: J7.2 6.81,34.91 R23.2
N$12
  Top 0.203: U1.45 17.13,7.98 17.53,8.38 17.53,9.02 17.97,9.46 C10.2 20,9.46 20.32,9.14 X2.2 20.32,8.25
N$13
  Top 0.203: U1.46 16.89,8.38 17.14,8.64 17.14,10.16 17.46,10.48 C12.2 20,10.48 20.32,10.79 X2.1
N$14
  Top 0.152: U1.37 16.81,4.78 17.4,4.19 X1.4 18.8,4.19 18.99,4 C1.1
N$15
  Top 0.152: X1.2 19.3,4.83 17.27,4.83 16.91,5.18 U1.38
  Top 0.203: C2.1 20.13,5.65 X1.2
N$16  (via drill 0.3 pad 0.64)
  Top 0.203: CDC.- v11.24,40.51 | U6.21 v3.56,28.96
  Bottom 0.203: v11.24,40.51 10.29,39.56 10.29,34.42 9.53,33.66 4.44,33.66 3.56,32.77 v3.56,28.96
N$17  (via drill 0.3 pad 0.64)
  Top 0.203: U7.HEAT v10.16,21.59
  other vias: 10.16,22.61
  pour Bottom (isolate 0.254): 9.02,23.37 11.56,23.37 11.56,20.57 9.02,20.57
N$19
  Top 0.152: C16.2 5.84,11.18 5.47,10.8 U2.10
N$20
  Top 0.152: U1.39 16.89,5.59 17.78,6.48 C6.1
N$21
  Top 0.203: U2.20 4.97,5.03 C17.2
N$25
  Top 0.203: U1.29 12.73,3.34 11.81,2.41 C7.1
N$26
  Top 0.203: U1.32 13.94,2.64 L2.2 C3.1
N$28
  Top 0.203: L3.2 L2.1 13.53,2.68 U1.31
N$29
  Top 0.203: C9.1 L3.1 12.38,2.48 13.13,3.23 U1.30
N$30
  Top 0.203: L1.1 C4.2 C3.2
N$31
  Top 0.203: L1.2 C5.2 ANT1.1
N$32
  Top 0.203: L5.1 13.78,13.02 L4.2
N$39
  Top 0.203: Q2.3 3.62,34.04 4.76,34.04 R21.2
N$40
  Top 0.406: J7.1 7.46,36.99 7.62,36.83
  Top 0.61: 7.62,36.83 7.62,35.43 F1.2
  pour Top (isolate 0.254, no thermals): 7.37,38.1 7.37,36.2 8.06,36.2 8.06,38.1
N$41
  Top 0.203: R20.2 R19.2 13.53,33.02 9.14,33.02 8.73,32.61 U6.9
N$42
  Top 0.203: R26.2 13.97,40 CDC.+
N$43
  Top 0.203: DAP.+ R25.2
N$44
  Top 0.203: R24.2 13.97,37.97 MSD.+
N$46  (via drill 0.3 pad 0.64)
  Top 0.203: U6.7 10.01,30.46 v10.67,31.11 | v11.24,37.46 MSD.-
  Bottom 0.203: v11.24,37.46 11.24,31.69 v10.67,31.11
N$47  (via drill 0.3 pad 0.64)
  Top 0.203: U6.12 7.23,32.63 v7.62,33.02 | DAP.- v11.24,38.99
  Bottom 0.203: v11.24,38.99 10.67,38.42 10.67,33.53 10.16,33.02 v7.62,33.02
N$78
  Top 0.203: D1.4 26.67,8.89 23.3,8.89 R4.1
N$79
  Top 0.305: U8.1 25.34,25.08 26.03,25.78 26.03,29.72 Q8.1
N$80
  Top 0.305: R39.2 U8.3
N$81
  Top 0.406: Q5.3 19.69,23.37 R37.2
N$82
  Top 0.406: Q4.3 22.99,23.11 R36.2
N$83
  Top 0.203: Q6.1 23.43,30.8 R41.2 R35.2
N$84
  Top 0.305: Q5.1 20.26,26.73 20.26,27.69 R33.2 20.13,28.26 19.69,28.7 Q7.3
N$85
  Top 0.203: Q7.1 20.13,30.8 R38.2 R42.2
N$86
  Top 0.203: R27.1 15.37,21.97 DONE.+
N$87
  Top 0.203: R28.1 CHRG.+
N$88
  Top 0.152: U1.40 16.84,5.98 17.97,7.11 21.4,7.11 R2.2
N$89
  Top 0.152: U1.41 16.8,6.38 17.84,7.43 21.84,7.43 21.91,7.37 R3.2
N$90
  Top 0.152: U1.42 16.75,6.78 17.72,7.75 21.27,7.75 R4.2
N$93
  Top 0.152: J1.2 2.92,5.78 2.92,13.08 3.81,13.97 10.6,13.97 11.18,13.4 11.18,11.56 11.94,10.8 U1.10
N$94
  Top 0.152: J1.3 2.6,8 2.6,13.21 3.68,14.29 10.73,14.29 11.49,13.52 11.49,11.68 12.33,10.84 U1.9
N$95
  Top 0.152: J1.4 2.29,10.22 2.29,13.33 3.56,14.6 10.86,14.6 11.81,13.65 11.81,11.81 12.73,10.89 U1.8
N$96
  Top 0.152: J1.5 1.27,12.76 3.43,14.92 10.99,14.92 12.13,13.78 12.13,11.94 13.13,10.93 U1.7
N$98
  Top 0.406: R39.1 C35.1 R36.1 R34.2 R37.1 R8.1
P12/SDA
  Top 0.203: U1.18 9.47,7.18 8.64,6.35 6.98,6.35 6.98,6.27 | 6.98,6.27 U2.24 | 6.98,6.27 6.98,5.21 R7.2
P13/SCL  (via drill 0.3 pad 0.64)
  Top 0.203: U1.19 9.58,6.78 8.51,5.71 v7.68,5.71 | U2.23 6.47,5.58 v6.4,5.51 5.97,5.08 R6.2
  Bottom 0.203: v6.4,5.51 7.48,5.51 v7.68,5.71
PROG-3V3  (via drill 0.3 pad 0.64)
  Top 0.203: v7.24,25.78 C24.1 7.23,25.28
  Top 0.254: U6.6 10.47,29.96 C23.1 | U6.29 7.23,25.28
  Top 0.305: R41.1 v21.91,31.75 | R24.1 R25.1 R26.1 v15.68,40.64 | 10.48,25.15 R18.2 v9.84,25.27 | v12.13,31.11 11.62,31.11 C23.1 | Q2.2 v1.59,32.38 | C26.2 v23.5,35.56 23.18,35.88 U5.2 | R42.1 18.54,32.77 v18.16,32.38
  pour POWER (isolate 0.254): 0,17.14 29.84,17.14 29.84,41.91 0,41.91
PROG-!CTS  (via drill 0.3 pad 0.64, 0.51 pad 0.76)
  Top 0.203: U1.14 9.88,8.78 9.65,9.02 9.65,9.78 v9.84,9.97 | U6.16 4.48,31.71 v4.44,31.75
  Bottom 0.203: v9.84,9.97 8.19,9.97 7.62,10.54 7.62,16.45 v7.68,16.51 7.62,16.57 7.62,19.05 4.44,22.22 v4.44,31.75
PROG-!RTS  (via drill 0.3 pad 0.64, 0.51 pad 0.76)
  Top 0.203: U1.16 9.67,7.98 8.89,8.76 8.89,10.67 v9.02,10.79 | U6.30 7.73,26.17 8.13,25.78 8.13,25.21 v8.25,25.08
  Bottom 0.203: v8.25,25.08 8.25,21.21 10.16,19.3 10.16,16.95 v9.72,16.51 9.02,15.81 v9.02,10.79
PROG-BUTTON  (via drill 0.3 pad 0.64)
  Top 0.203: U6.3 10.28,28.46 v10.54,28.19 | v5.72,22.92 4.99,22.92 | SW2.4 SW2.3 4.95,22.91 | 4.99,22.92 4.99,22.91 4.95,22.91 | 4.95,22.91 4.95,22.86 5.08,22.86 5.08,22.99 4.95,22.99 4.95,22.92 | 4.99,22.92 4.95,22.92 | 4.95,22.92 4.95,22.91
  Bottom 0.203: v10.54,28.19 9.02,26.67 6.35,26.67 5.72,26.03 v5.72,22.92
PROG-RESET
  Top 0.203: U6.2 9.92,27.96 10.48,27.41 R18.1 C22.2
PROG-RX  (via drill 0.3 pad 0.64, 0.51 pad 0.76)
  Top 0.203: U1.15 9.78,8.38 9.27,8.89 9.27,10.22 v9.84,10.79 9.78,10.73 | U6.31 8.23,26.25 v8.89,25.59
  Bottom 0.203: v8.89,25.59 8.89,21.21 11.43,18.67 J5.2 11.43,17.21 v10.73,16.51 9.84,15.62 v9.84,10.79
PROG-TX  (via drill 0.3 pad 0.64, 0.51 pad 0.76)
  Top 0.203: U1.17 9.56,7.58 8.51,8.64 8.51,10.48 v8.19,10.79 | U6.32 8.73,26.63 8.99,26.63 v9.46,26.16
  Bottom 0.203: v9.46,26.16 8.47,26.16 7.62,25.31 7.62,19.68 J5.1 8.89,16.7 v8.7,16.51 8.19,16 v8.19,10.79
PROG-VCC  (via drill 0.3 pad 0.64)
  Top 0.406: 21.34,25.4 19.81,25.4 Q5.2 18.8,27.69 | 21.34,25.4 22.1,26.16 Q4.2 21.97,26.54 v21.97,27.69 | 21.34,25.4 21.34,23.24 R34.1 | R29.1 v26.67,29.02 | Q3.P1 18.27,36.43 Q3.6 v17.4,35.56 C31.2 | Q3.4 16.88,37.73 v16.51,38.1 | 18.8,27.69 v18.41,27.69 | R33.1 18.8,27.69 | R32.2 v21.97,27.69 | v21.97,27.69 C32.1
  POWER 0.406: v16.51,38.1 15.88,37.46 15.88,36.2 16.51,35.56 v17.4,35.56 17.4,28.7 v18.41,27.69 | v26.67,29.02 23.3,29.02 v21.97,27.69
  Bottom 0.61: P-VCC.T 16.51,34.67 v17.4,35.56
PRPH-3V3  (via drill 0.3 pad 0.64)
  Top 0.203: 15.88,14.29 C21.1
  Top 0.254: U3.6 15.69,14.1 C21.1 v16.32,14.1
  POWER 0.254: v16.32,14.1 15.11,15.3 2.29,15.3 J1.6
PRPH-PWR-CTL  (via drill 0.3 pad 0.64)
  Top 0.203: U1.3 14.73,11.24 v14.54,11.43 | U3.1 v19.01,13.33 19.01,12.74 19.05,12.7 R12.2
  Bottom 0.203: v19.01,13.33 19.01,11.58 18.22,10.79 15.18,10.79 v14.54,11.43
VBAT_SENSE  (via drill 0.3 pad 0.64)
  Top 0.203: 12.95,12.19 C14.1 13.94,11.02 v13.94,10.79 U1.5 | R14.1 v21.34,13.33 21.34,12.76 R17.2
  Bottom 0.203: v13.94,10.79 14.32,10.41 18.41,10.41 v21.34,13.33
VCC  (via drill 0.3 pad 0.64, 0.51 pad 0.76)
  Top 0.406: BAT1.+ v24.7,12.19 24.7,14.41 24.13,14.99 R14.2 20.45,14.99 | 20.45,14.99 C19.2 20.07,14.99 | 20.33,15.1 20.45,14.99 | U3.2 19.01,14.99 | 19.01,14.99 U3.3 | 20.07,14.99 19.01,14.99 | R8.2 18.03,21.72 18.03,19.43 J9.2 19.88,17.59 v19.88,16.51 19.88,15.18 20.07,14.99
  Bottom 0.203: 25.78,12.19 25.91,12.19 BAT+.1
  Bottom 0.406: v24.7,12.19 25.78,12.19 | J9.1 J9.2
VUSB  (via drill 0.3 pad 0.64)
  Top 0.203: C34.2 7.43,21.21 7.44,21.22
  Top 0.305: 7.44,21.22 U7.4 8.75,21.1 8.76,21.08 | U8.5 v25.34,27.56 C33.1
  Top 0.406: R19.1 C27.2 11.75,34.73 11.68,34.67 11.68,34.42 F1.1 11.56,34.16 11.81,34.42 11.81,34.48 | 8.76,21.08 8.76,20.65 9.22,20.19 16.64,20.19 17.21,20.76 R31.1 v17.21,21.47 R27.2 R28.2 v17.21,24.13 | R19.1 14.35,34.8 | Q3.5 v16.57,37.08 15.24,37.08 v14.41,36.26 14.35,36.2 R19.1 | Q3.1 19.49,36.37 19.49,35.18 19.56,35.18 19.81,34.92 U5.3 19.7,34.73 C25.2 v18.41,35.56
  POWER 0.406: v17.21,24.13 16.64,24.7 16.64,34.04 v14.41,36.26 | v16.57,37.08 17.53,37.08 18.41,36.2 v18.41,35.56 | v17.21,21.47 22.1,21.47 25.34,24.7 v25.34,27.56
  Bottom 0.61: VUSB.T 13.97,35.81 v14.41,36.26

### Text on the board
tPlace: CHRG | - | chrg | + | done | X | Z | Y | BAT
bPlace: SWDIO | SWCLK | RxD | TxD | VCC | VCC | GND | GND | OUT_3V3 | P3 | 3.5-4.2V | P4 | BLE Smurfs | P5 | v1.0 10/30/2014 | P6 | by Seeed Studio | GND | www.seeedstudio.com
